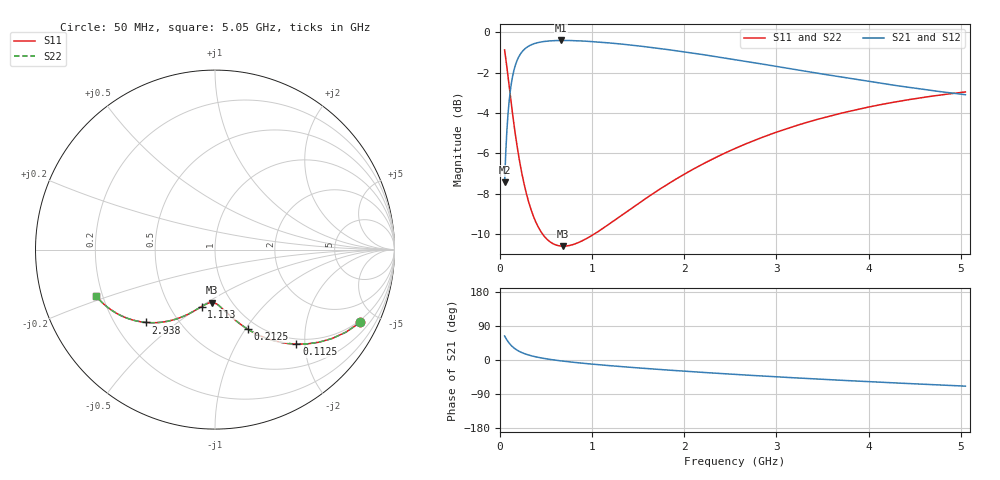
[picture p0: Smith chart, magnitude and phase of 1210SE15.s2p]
! AVX Thin Film Operation		Date: August 2001
! Description: Accu-P® Series, Thin Film, SMD, RF Capacitor
! Part Number: 12101J150FBT
! 50 MHz  -  5.05 GHz
! Serial Measurements
# mhz S db R 50
!	S11		S21		S12		S22
!	dB	Phase	dB	Phase	dB	Phase	dB	Phase
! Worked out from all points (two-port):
!   401 points, 50 MHz to 5.05 GHz, reference 50 ohm
!   highest |S21| = -0.40 dB at 662.5 MHz (marker M1); lowest = -7.4 dB at 50 MHz (marker M2)
!   |S21| within 3 dB of the highest: 99.45 MHz to end of sweep
!   lowest |S11| = -10.6 dB at 687.5 MHz (marker M3), VSWR 1.84, Z = 40.8 - j26.4 ohm
!   |S11| at or under -10 dB: 462.7 MHz to 1.02 GHz (557.3 MHz wide, 75.2 % of centre)
!   |S22| runs from -10.6 to -0.9 dB; largest |S21 - S12| = 0
!   S11 on the Smith chart (normalised r, x): 50 MHz: 0.90, -4.04; 112.5 MHz: 0.90, -1.83; 212.5 MHz: 0.89, -1.03; 1.113 GHz: 0.71, -0.51; 2.938 GHz: 0.33, -0.39; 5.05 GHz: 0.17, -0.18
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50  -0.87 -26.6  -7.43 63.4  -7.43 63.4  -0.87 -26.6
62.5  -1.28 -32.2  -5.95 57.8  -5.95 57.8  -1.28 -32.2
87.5  -2.20 -41.7  -4.01 48.3  -4.01 48.3  -2.20 -41.7
112.5  -3.16 -49.3  -2.87 40.7  -2.87 40.7  -3.16 -49.3
137.5  -4.08 -55.4  -2.16 34.6  -2.16 34.6  -4.08 -55.4
162.5  -4.93 -60.3  -1.69 29.7  -1.69 29.7  -4.93 -60.3
212.5  -6.38 -67.6  -1.14 22.4  -1.14 22.4  -6.38 -67.6
287.5  -8.01 -75.1  -0.75 14.9  -0.75 14.9  -8.01 -75.1
400  -9.51 -82.3  -0.52 7.7  -0.52 7.7  -9.51 -82.3
525  -10.31 -87.7  -0.43 2.2  -0.43 2.2  -10.31 -87.7
662.5  -10.59 -92.3  -0.40 -2.3  -0.40 -2.3  -10.59 -92.3
687.5  -10.60 -93.0  -0.40 -3.1  -0.40 -3.1  -10.60 -93.0
887.5  -10.34 -98.3  -0.42 -8.3  -0.42 -8.3  -10.34 -98.3
1112.5  -9.72 -103.3  -0.49 -13.3  -0.49 -13.3  -9.72 -103.3
1412.5  -8.76 -109.2  -0.62 -19.3  -0.62 -19.3  -8.76 -109.2
1725  -7.79 -114.9  -0.79 -24.9  -0.79 -24.9  -7.79 -114.9
2125  -6.71 -121.5  -1.05 -31.5  -1.05 -31.5  -6.71 -121.5
2550  -5.75 -128.0  -1.35 -38.0  -1.35 -38.0  -5.75 -128.0
2937.5  -5.05 -133.5  -1.64 -43.5  -1.64 -43.5  -5.05 -133.5
3387.5  -4.38 -139.5  -1.98 -49.5  -1.98 -49.5  -4.38 -139.5
4225  -3.50 -149.7  -2.58 -59.8  -2.58 -59.8  -3.50 -149.7
5050  -2.95 -158.9  -3.09 -69.0  -3.09 -69.0  -2.95 -158.9
